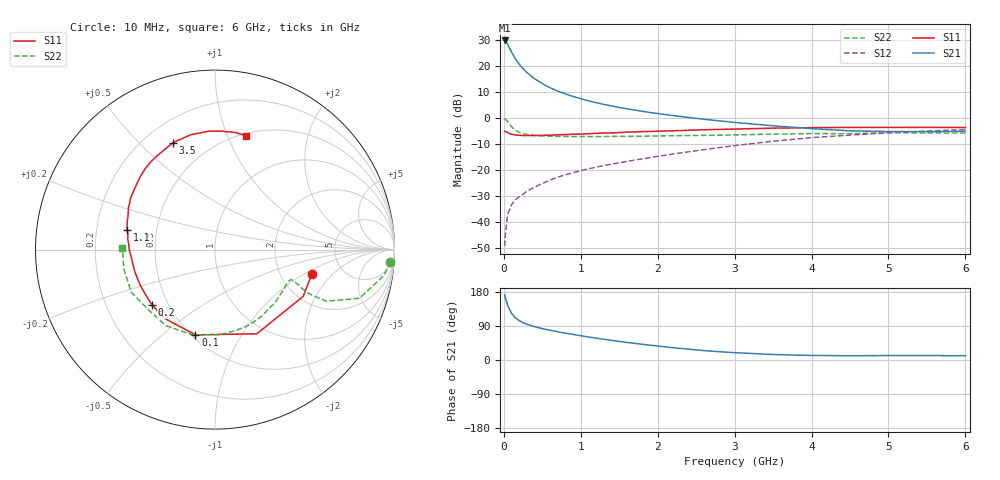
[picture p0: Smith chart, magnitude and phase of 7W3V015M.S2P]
! Infineon Technologies  Discrete & RF Semiconductors
! BFS17W
! Si NPN RF Bipolar Junction Transistor in SOT323
! VCE = 3 V  IC = 15 mA
! Common Emitter S-Parameters:  August  1999
# GHz  S  MA  R  50
!  f  S11  S21  S12  S22
! GHz  MAG  ANG  MAG  ANG  MAG  ANG  MAG  ANG
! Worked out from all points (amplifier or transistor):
!   36 points, 10 MHz to 6 GHz, reference 50 ohm
!   highest |S21| = 29.7 dB at 10 MHz (marker M1)
!   |S21| within 3 dB of that: start of sweep to 75.2 MHz
!   unconditionally stable (mu >= 1): 325.5 MHz to 2.446 GHz; 4.451 GHz to end of sweep
!   at 250 MHz: K = 0.92, MSG = 24.0 dB, |S12| = -29.2 dB
!   at 1.4 GHz: K = 1.20, MAG = 8.4 dB, |S12| = -17.7 dB
!   at 6 GHz: K = 1.07, MAG = -1.9 dB, |S12| = -4.4 dB
!   S11 on the Smith chart (normalised r, x): 10 MHz: 3.00, -1.18; 100 MHz: 0.52, -0.65; 200 MHz: 0.41, -0.32; 1.1 GHz: 0.34, +0.10; 3.5 GHz: 0.31, +0.64; 6 GHz: 0.52, +1.16
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0.01  0.5566 -14.1  30.68 172.3  0.0035 80.4  0.9793 -4.0
0.02  0.5563 -27.9  29.92 164.2  0.006 83.4  0.9521 -8.7
0.05  0.5237 -63.6  25.69 144.1  0.0143 69.4  0.8498 -18.6
0.1  0.4874 -102.9  18.42 123.4  0.0219 57.2  0.6825 -24.9
0.15  0.4745 -125.7  13.7 111.3  0.0271 55.4  0.5838 -25.2
0.2  0.4674 -138.8  10.78 104.0  0.031 56.8  0.5328 -24.1
0.25  0.4606 -148.3  8.815 98.6  0.0347 58.2  0.5013 -22.8
0.3  0.4615 -154.7  7.443 94.5  0.0396 59.8  0.4848 -22.1
0.4  0.4632 -164.5  5.67 87.9  0.0476 62.8  0.4628 -21.5
0.5  0.4652 -170.6  4.57 82.9  0.0555 64.5  0.4546 -21.6
0.6  0.469 -175.5  3.818 78.5  0.0646 66.2  0.4492 -22.4
0.7  0.4771 -179.6  3.298 74.5  0.0736 66.7  0.4449 -23.9
0.9  0.4892 173.4  2.589 67.4  0.0895 68.2  0.4415 -27.5
1.1  0.5011 167.2  2.14 60.7  0.1064 68.6  0.442 -32.0
1.3  0.5149 161.4  1.827 54.6  0.123 68.6  0.4419 -37.2
1.6  0.5367 153.9  1.501 46.3  0.1475 69.1  0.4447 -45.2
2.2  0.5695 139.9  1.116 32.5  0.2044 69.1  0.4583 -63.2
2.8  0.6055 126.2  0.883 21.9  0.2709 66.3  0.4696 -82.4
3.5  0.6403 111.4  0.71 14.5  0.3596 60.3  0.4915 -105.1
4.5  0.6603 93.1  0.569 11.3  0.4706 47.6  0.5007 -138.9
5.5  0.6621 80.0  0.546 11.8  0.5633 35.0  0.5188 -167.9
6  0.6577 75.0  0.557 11.2  0.5999 28.9  0.5168 179.3
